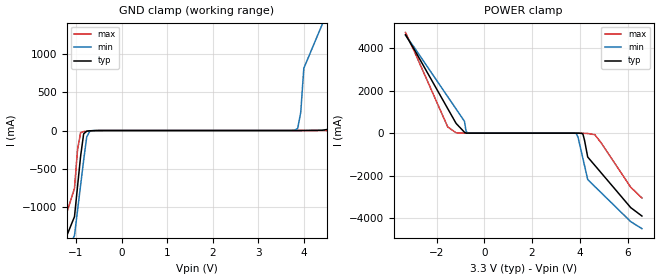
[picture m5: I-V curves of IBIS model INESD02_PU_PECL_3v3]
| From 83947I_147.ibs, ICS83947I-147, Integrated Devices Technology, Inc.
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[Model] INESD02_PU_PECL_3v3
Model_type  Input
Polarity   Non-Inverting
Vinl = 0.8V
Vinh = 2.0V
|   typ   min   max
C_comp   2pF   1.5pF   2.5pF
|   typ   min   max
[Voltage range]  3.3V   3.15V   3.45V
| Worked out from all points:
|   GND clamp passes 1 mA (typ) near -0.59 V on its own axis
|   POWER clamp passes 1 mA (typ) near -0.70 V on its own axis
[GND_clamp]
|Voltage   I(typ)   I(min)   I(max)
-3.3V     -3.894A    -3.674A    -4.294A
-1.3V     -1.521A    -1.7A      -1.261A
-1.031V   -1.125A    -1.372A    -755.3mA
-896.9mV  -335.4mA   -714.7mA   -27.07mA
-695.9mV  -3.401mA   -10.69mA   -6.477mA
3.794V    17.99uA    3.319mA    6.081uA
3.928V    181.1uA    239mA      10.12uA
3.995V    711.6uA    813.7mA    20.78uA
4.8V      40.44mA    1.967A     268.6uA
5.6V      1.139A     3.12A      2.243mA
6.3V      2.525A     4.275A     64.01mA
6.6V      3.219A     4.852A     752.7mA
[POWER_clamp]
|Voltage   I(typ)   I(min)   I(max)
-3.3V     4.617A     4.594A     4.726A
-1.53V    1.149A     1.709A     289.6mA
-1.18V    456.4mA    1.132A     15.33mA
-829.9mV  42.02mA    556.1mA    3.39mA
-762.9mV  4.159mA    91mA       1.422mA
-695.9mV  727.9uA    10.66mA    491.6uA
3.861V    -620.9uA   -26.2mA    -103.4uA
4.129V    -41.91mA   -1.19A     -4.968mA
4.33V     -1.119A    -2.176A    -17.93mA
4.63V     -1.515A    -2.505A    -71.45mA
6.13V     -3.492A    -4.151A    -2.536A
6.6V      -3.888A    -4.48A     -3.041A
